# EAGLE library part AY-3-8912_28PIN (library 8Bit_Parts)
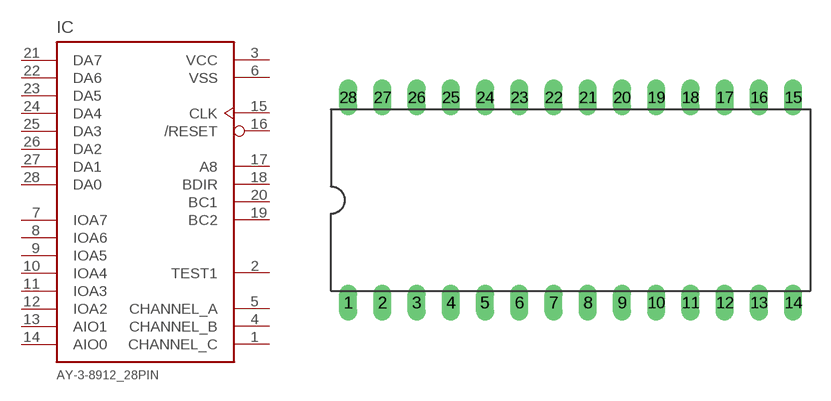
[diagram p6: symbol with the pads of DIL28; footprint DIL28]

Designator prefix IC

## AY-3-8912_28PIN  [DIL28]
1  CHANNEL_C  out
2  TEST1  nc
3  VCC  pwr
4  CHANNEL_B  out
5  CHANNEL_A  out
6  VSS  pwr
7  IOA7
8  IOA6
9  IOA5
10  IOA4
11  IOA3
12  IOA2
13  AIO1
14  AIO0
15  CLK  in
16  /RESET  in
17  A8  in
18  BDIR  in
19  BC2  in
20  BC1  in
21  DA7
22  DA6
23  DA5
24  DA4
25  DA3
26  DA2
27  DA1
28  DA0

## Footprint DIL28 (pad centres in mm)
Dual In Line Package
drill 0.813 long: 1 -16.51,-7.62; 2 -13.97,-7.62; 3 -11.43,-7.62; 4 -8.89,-7.62; 5 -6.35,-7.62; 6 -3.81,-7.62; 7 -1.27,-7.62; 8 1.27,-7.62; 9 3.81,-7.62; 10 6.35,-7.62; 11 8.89,-7.62; 12 11.43,-7.62; 13 13.97,-7.62; 14 16.51,-7.62; 15 16.51,7.62; 16 13.97,7.62; 17 11.43,7.62; 18 8.89,7.62; 19 6.35,7.62; 20 3.81,7.62; 21 1.27,7.62; 22 -1.27,7.62; 23 -3.81,7.62; 24 -6.35,7.62; 25 -8.89,7.62; 26 -11.43,7.62; 27 -13.97,7.62; 28 -16.51,7.62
